(* Logix 5000 Routine export IS7800_Trigger; software revision 33.01 *)

VAR_GLOBAL   (* controller tags *)
   Enable : BOOL := 1;
   Job_Change_In_Process : BOOL;
   Timer : TIMER := (PRE := 1000);
   Timer1 : TIMER := (PRE := 65);   // Hold Longer than RPI of AOP.
   TimerTriggerCMD : BOOL;
   TriggerCMD : BOOL;
END_VAR

PROGRAM MainProgram

ROUTINE IS7800_Trigger   (* ladder *)
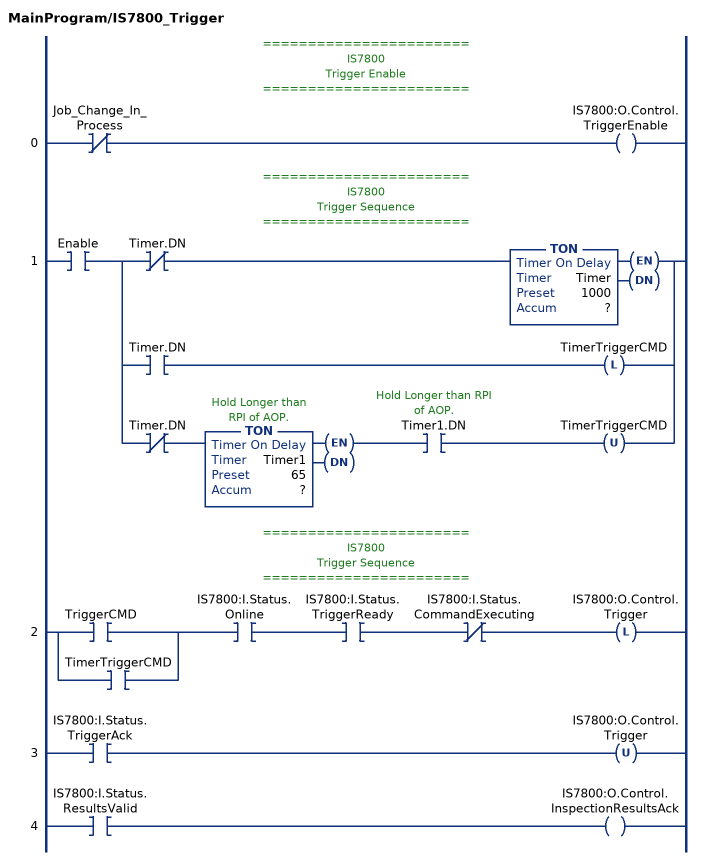
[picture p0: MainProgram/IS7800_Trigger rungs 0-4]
   // =======================
   // IS7800
   // Trigger Enable
   // =======================
   0: XIO(Job_Change_In_Process)OTE(IS7800:O.Control.TriggerEnable);
   // =======================
   // IS7800
   // Trigger Sequence
   // =======================
   1: XIC(Enable)[XIO(Timer.DN) TON(Timer,?,?) ,XIC(Timer.DN) OTL(TimerTriggerCMD) ,XIO(Timer.DN) TON(Timer1,?,?) XIC(Timer1.DN) OTU(TimerTriggerCMD) ];
   // =======================
   // IS7800
   // Trigger Sequence
   // =======================
   2: [XIC(TriggerCMD) ,XIC(TimerTriggerCMD) ]XIC(IS7800:I.Status.Online)XIC(IS7800:I.Status.TriggerReady)XIO(IS7800:I.Status.CommandExecuting)OTL(IS7800:O.Control.Trigger);
   3: XIC(IS7800:I.Status.TriggerAck)OTU(IS7800:O.Control.Trigger);
   4: XIC(IS7800:I.Status.ResultsValid)OTE(IS7800:O.Control.InspectionResultsAck);
END_ROUTINE
END_PROGRAM
